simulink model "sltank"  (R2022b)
settings: Solver=ode45  StartTime=0  StopTime=10000  MaxStep=0.2  RelTol=1e-3  AbsTol=1e-6
PreLoadFcn:
  | tank = readfis('tank');
libraries: fuzblock x1, slpidlib x1

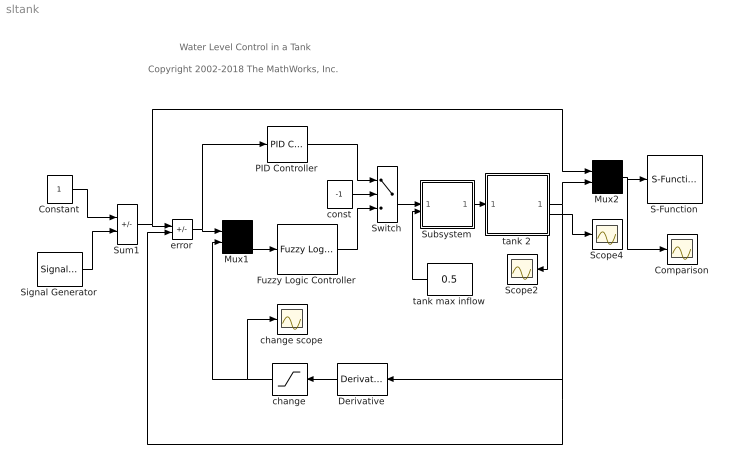
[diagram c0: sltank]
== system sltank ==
  note: Copyright 2002-2018 The MathWorks, Inc.
  note: Water Level Control in a Tank
  Comparison : Scope
  Constant : Constant
  Derivative : Derivative
  Fuzzy Logic Controller : fuzblock/Fuzzy Logic  Controller  FIS=tank  OutputSampleNumber=101  DataType=double  FuzzifiedInputs=off  RuleFiringStrengths=off  RuleOutputs=off  AggregatedOutputs=off  SimulateUsing=Interpreted execution  OutOfRangeInputValueMessage=warning  NoRuleFiredMessage=warning  EmptyOutputFuzzySetMessage=warning
  Mux1 : Mux  Inputs=2
  Mux2 : Mux  Inputs=2
  PID Controller : slpidlib/PID Controller  Controller=PID  Form=Parallel  TimeDomain=Continuous-time  UseExternalTs=off  SampleTime=1  IntegratorMethod=Forward Euler  FilterMethod=Forward Euler  ControllerParametersSource=internal  P=2  I=0  UseKiTs=off  D=1  N=100  UseFilter=on  TunerSelectOption=Transfer Function Based (PID Tuner App)  InitialConditionSource=internal  InitialConditionForIntegrator=0  InitialConditionForFilter=0  DifferentiatorICPrevScaledInput=0  ExternalReset=none  TrackingMode=off  Kt=1  LimitOutput=off  SatLimitsSource=internal  UpperSaturationLimit=inf  LowerSaturationLimit=-inf  LinearizeAsGain=off  AntiWindupMode=none  Kb=1  LimitIntegrator=off  UpperIntegratorSaturationLimit=inf  LowerIntegratorSaturationLimit=-inf  POutMin=[]  POutMax=[]  IOutMin=[]  IOutMax=[]  DOutMin=[]  DOutMax=[]  NOutMin=[]  NOutMax=[]  SumOutMin=[]  SumOutMax=[]  SaturationOutMin=[]  SaturationOutMax=[]  PParamMin=[]  PParamMax=[]  IParamMin=[]  IParamMax=[]  DParamMin=[]  DParamMax=[]  NParamMin=[]  NParamMax=[]  KbParamMin=[]  KbParamMax=[]  KtParamMin=[]  KtParamMax=[]  KbOutMin=[]  KbOutMax=[]  KtOutMin=[]  KtOutMax=[]  IntegratorOutMin=[]  IntegratorOutMax=[]  FilterOutMin=[]  FilterOutMax=[]  SumI1OutMin=[]  SumI1OutMax=[]  SumI2OutMin=[]  SumI2OutMax=[]  SumI3OutMin=[]  SumI3OutMax=[]  SumI4OutMin=[]  SumI4OutMax=[]  SumDOutMin=[]  SumDOutMax=[]  DifferentiatorOutMin=[]  DifferentiatorOutMax=[]  FilterDiffOutCoefMin=[]  FilterDiffOutCoefMax=[]  ReciprocalOutMin=[]  ReciprocalOutMax=[]  SumDenOutMin=[]  SumDenOutMax=[]  SumNumOutMin=[]  SumNumOutMax=[]  DivideOutMin=[]  DivideOutMax=[]  UdiffTsProdOutMin=[]  UdiffTsProdOutMax=[]  NTsProdOutMin=[]  NTsProdOutMax=[]  UintegralTsProdOutMin=[]  UintegralTsProdOutMax=[]  UngainTsProdOutMin=[]  UngainTsProdOutMax=[]  IntegratorContinuousStateAttributes=''  IntegratorStateMustResolveToSignalObject=off  IntegratorRTWStateStorageClass=Auto  FilterContinuousStateAttributes=''  FilterStateMustResolveToSignalObject=off  FilterRTWStateStorageClass=Auto  ParallelPVariant=InternalParameters  IdealPVariant=Disabled  IVariant=InternalParameters  DVariant=InternalParameters  IntegratorVariant=Continuous  SatVariant=Disabled  AWVariant=Passthrough  PCopyVariant=Disabled  TRVariant=Disabled  FdbkBlocksVariant=Forward  IdealPFdbkVariant=Disabled  SatFdbkVariant=Disabled  DerivativeFilterVariant=ContFilter  NVariant=InternalParameters  NCopyVariant=Disabled  FilterICVariant=InternalICsFilter  IntegratorICVariant=InternalICs  ExternalResetVariant=Disabled  TRSumVariant=Passthrough  SumFdbkVariant=Disabled  SumVariant=Sum_PID  TsampFilterVariant=InternalTs  TsampNgainVariant=Passthrough  TsampIntegralVariant=Passthrough  ExternalSaturationOutDataTypeStr=Inherit: Same as second input
  S-Function : S-Function  FunctionName=animtank  Parameters=1  SFunctionDeploymentMode=off  EnableBusSupport=off
  Scope2 : Scope
  Scope4 : Scope
  Signal Generator : SignalGenerator  WaveForm=square  Amplitude=0.500000  Frequency=0.100000  Units=rad/sec
  Subsystem : Subsystem  mask(Valve){InitialPosition=0}
      mask prompts: InitialPosition "Initial position [0=closed 1=open]:"
      mask help: Valve
  Sum1 : Sum  Inputs=+-  InputSameDT=on  SaturateOnIntegerOverflow=on
  Switch : Switch
  change : Saturate  UpperLimit=0.1  LowerLimit=-0.1
  change scope : Scope
  const : Constant  Value=-1
  error : Sum  Inputs=+-  InputSameDT=on  SaturateOnIntegerOverflow=on
  tank 2 : Subsystem  mask(Water tank){ht=2, area=1, outletArea=0.05, overflowLimit=0, initialHt=0.5}
      mask prompts: ht "Height of tank (m):"; area "Bottom area (m^2):"; outletArea "Out pipe crossection (m^2):"; overflowLimit "Overflow sensor distance from top (m):"; initialHt "Initial level height (m):"
      mask help: Cylindrical water tank with overflow signal
  tank max inflow : Constant  Value=0.5
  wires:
  tank 2/2(flow out) -> Scope4/1
  tank max inflow/1 -> Subsystem/2(source flow)
  Derivative/1 -> change/1
  Mux1/1 -> Fuzzy Logic Controller/1
  change/1 -> Mux1/2, change scope/1
  Constant/1 -> Sum1/1
  Signal Generator/1 -> Sum1/2
  Subsystem/1(out flow) -> tank 2/1(flow in)
  tank 2/1(water level) -> Mux2/2, error/2, Derivative/1
  Sum1/1 -> error/1, Mux2/1
  tank 2/3(overflow flag) -> Scope2/1
  Switch/1 -> Subsystem/1(control)
  Mux2/1 -> S-Function/1, Comparison/1
  error/1 -> Mux1/1, PID Controller/1
  Fuzzy Logic Controller/1 -> Switch/3
  PID Controller/1 -> Switch/1
  const/1 -> Switch/2

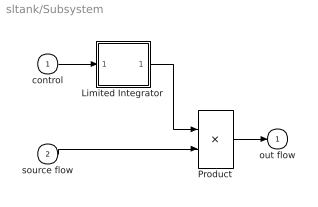
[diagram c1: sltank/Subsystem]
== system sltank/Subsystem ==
  control : Inport
  source flow : Inport  Port=2
  Limited Integrator : Subsystem  mask(Limited integrator.){lb=0, ub=1, xi=InitialPosition}
      mask prompts: lb "Lower bound:"; ub "Upper bound:"; xi "Initial condition"
      mask help: Limited integrator
  Product : Product  InputSameDT=on  RndMeth=Zero  SaturateOnIntegerOverflow=on
  out flow : Outport  InitialOutput=0  VectorParamsAs1DForOutWhenUnconnected=off
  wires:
  source flow/1 -> Product/2
  Product/1 -> out flow/1
  control/1 -> Limited Integrator/1(In_1)
  Limited Integrator/1(Out_1) -> Product/1

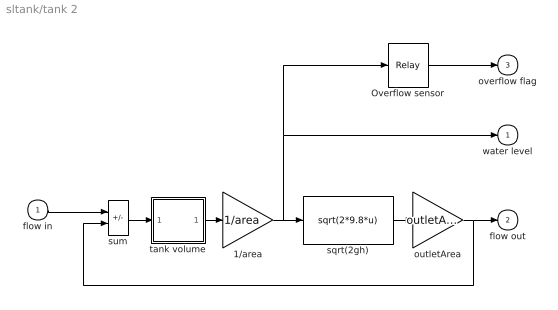
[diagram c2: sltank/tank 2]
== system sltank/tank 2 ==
  flow in : Inport
  1/area : Gain  Gain=1/area  SaturateOnIntegerOverflow=on
  Overflow sensor : Relay  OnSwitchValue=ht - overflowLimit  OffSwitchValue=ht - overflowLimit
  outletArea : Gain  Gain=outletArea  SaturateOnIntegerOverflow=on
  sqrt(2gh) : Fcn  Expr=sqrt(2*9.8*u)
  sum : Sum  Inputs=+-  InputSameDT=on  SaturateOnIntegerOverflow=on
  tank volume : Subsystem  mask(Limited integrator.){lb=0, ub=ht * area, xi=initialHt * area}
      mask prompts: lb "Lower bound:"; ub "Upper bound:"; xi "Initial condition"
      mask help: Limited integrator
  water level : Outport  InitialOutput=0  VectorParamsAs1DForOutWhenUnconnected=off
  flow out : Outport  Port=2  InitialOutput=0  VectorParamsAs1DForOutWhenUnconnected=off
  overflow flag : Outport  Port=3  InitialOutput=0  VectorParamsAs1DForOutWhenUnconnected=off
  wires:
  outletArea/1 -> flow out/1, sum/2
  sqrt(2gh)/1 -> outletArea/1
  1/area/1 -> Overflow sensor/1, water level/1, sqrt(2gh)/1
  tank volume/1(Out_1) -> 1/area/1
  Overflow sensor/1 -> overflow flag/1
  flow in/1 -> sum/1
  sum/1 -> tank volume/1(In_1)

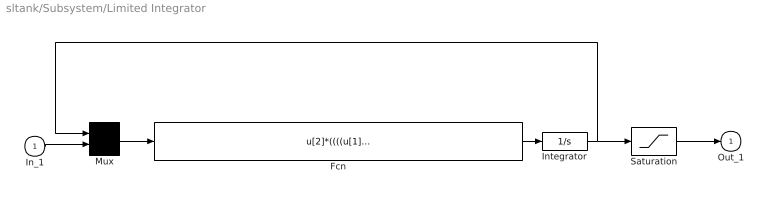
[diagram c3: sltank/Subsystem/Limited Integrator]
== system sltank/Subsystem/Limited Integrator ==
  In_1 : Inport
  Fcn : Fcn  Expr=u[2]*((((u[1]>lb)+(u[2]>=0))>0) * (((u[1]<ub)+(u[2]<=0))>0))
  Integrator : Integrator  InitialCondition=xi
  Mux : Mux  Inputs=2
  Saturation : Saturate  UpperLimit=ub  LowerLimit=lb
  Out_1 : Outport  InitialOutput=0  VectorParamsAs1DForOutWhenUnconnected=off
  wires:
  Integrator/1 -> Saturation/1, Mux/1
  Fcn/1 -> Integrator/1
  Mux/1 -> Fcn/1
  In_1/1 -> Mux/2
  Saturation/1 -> Out_1/1

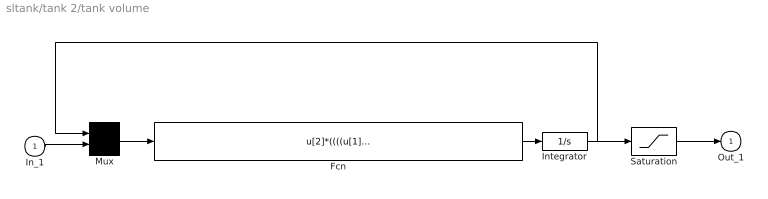
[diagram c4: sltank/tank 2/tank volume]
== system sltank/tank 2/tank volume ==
  In_1 : Inport
  Fcn : Fcn  Expr=u[2]*((((u[1]>lb)+(u[2]>=0))>0) * (((u[1]<ub)+(u[2]<=0))>0))
  Integrator : Integrator  InitialCondition=xi
  Mux : Mux  Inputs=2
  Saturation : Saturate  UpperLimit=ub  LowerLimit=lb
  Out_1 : Outport  InitialOutput=0  VectorParamsAs1DForOutWhenUnconnected=off
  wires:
  Integrator/1 -> Saturation/1, Mux/1
  Fcn/1 -> Integrator/1
  Mux/1 -> Fcn/1
  In_1/1 -> Mux/2
  Saturation/1 -> Out_1/1
